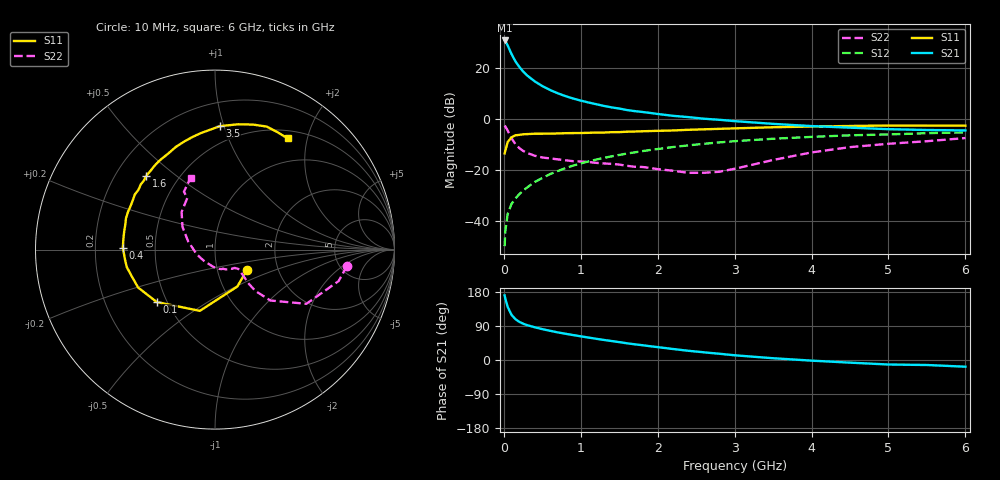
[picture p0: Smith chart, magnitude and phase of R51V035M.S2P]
! SIEMENS Small Signal Semiconductors
! BFR183
! Si NPN RF Bipolar Junction Transistor in SOT23
! VCE = 1 V  IC = 35 mA
! Common Emitter S-Parameters:  May  1996
# GHz  S  MA  R  50
!  f  S11  S21  S12  S22
! GHz  MAG  ANG  MAG  ANG  MAG  ANG  MAG  ANG
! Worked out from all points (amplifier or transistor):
!   36 points, 10 MHz to 6 GHz, reference 50 ohm
!   highest |S21| = 30.8 dB at 10 MHz (marker M1)
!   |S21| within 3 dB of that: start of sweep to 65.29 MHz
!   unconditionally stable (mu >= 1): start of sweep to 23.88 MHz; 168.8 MHz to end of sweep
!   at 250 MHz: K = 1.11, MAG = 21.4 dB, |S12| = -28.1 dB
!   at 1.4 GHz: K = 1.19, MAG = 7.0 dB, |S12| = -14.7 dB
!   at 6 GHz: K = 1.05, MAG = -0.9 dB, |S12| = -5.3 dB
!   S11 on the Smith chart (normalised r, x): 10 MHz: 1.39, -0.33; 100 MHz: 0.44, -0.32; 400 MHz: 0.32, +0.01; 1.6 GHz: 0.33, +0.40; 3.5 GHz: 0.37, +0.97; 6 GHz: 0.61, +1.68
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0.01  0.2114 -32.3  34.63 170.5  0.0032 74.6  0.7416 -7.0
0.02  0.2405 -58.9  33.48 161.5  0.0065 76.0  0.7106 -14.3
0.05  0.3517 -103.9  27.6 139.9  0.0137 66.3  0.5918 -30.7
0.1  0.4366 -138.0  18.73 119.2  0.0216 63.0  0.4189 -42.6
0.15  0.4779 -153.8  13.53 107.7  0.0275 63.1  0.3211 -45.7
0.2  0.4873 -162.4  10.56 100.8  0.0333 65.0  0.269 -45.3
0.25  0.5008 -168.7  8.551 95.9  0.0392 66.8  0.2368 -44.0
0.3  0.5042 -173.4  7.186 92.2  0.045 68.7  0.2164 -42.9
0.4  0.5134 178.7  5.477 86.5  0.0579 70.2  0.1903 -41.0
0.5  0.5138 173.7  4.416 81.5  0.0695 70.7  0.1755 -39.8
0.6  0.5159 168.8  3.703 77.1  0.0828 70.6  0.1682 -39.8
0.7  0.5191 164.1  3.191 72.9  0.0951 70.1  0.1615 -40.7
0.9  0.5284 156.4  2.518 65.8  0.1217 68.4  0.1487 -43.3
1.1  0.5347 148.8  2.104 59.2  0.1469 66.4  0.1432 -48.3
1.3  0.541 142.1  1.804 52.9  0.1724 63.9  0.1341 -53.0
1.6  0.5623 132.8  1.496 44.1  0.2095 59.9  0.1206 -64.3
2.2  0.5946 116.2  1.152 29.0  0.2814 51.1  0.0966 -96.2
2.8  0.6398 101.3  0.963 16.5  0.3467 41.8  0.0922 -149.3
3.5  0.688 87.8  0.801 4.7  0.409 30.4  0.1567 162.9
4.5  0.728 73.1  0.675 -7.0  0.4779 16.2  0.2803 131.6
5.5  0.741 61.7  0.607 -13.2  0.5262 4.4  0.3661 118.2
6  0.7399 56.9  0.596 -17.7  0.5455 -2.8  0.422 108.8
